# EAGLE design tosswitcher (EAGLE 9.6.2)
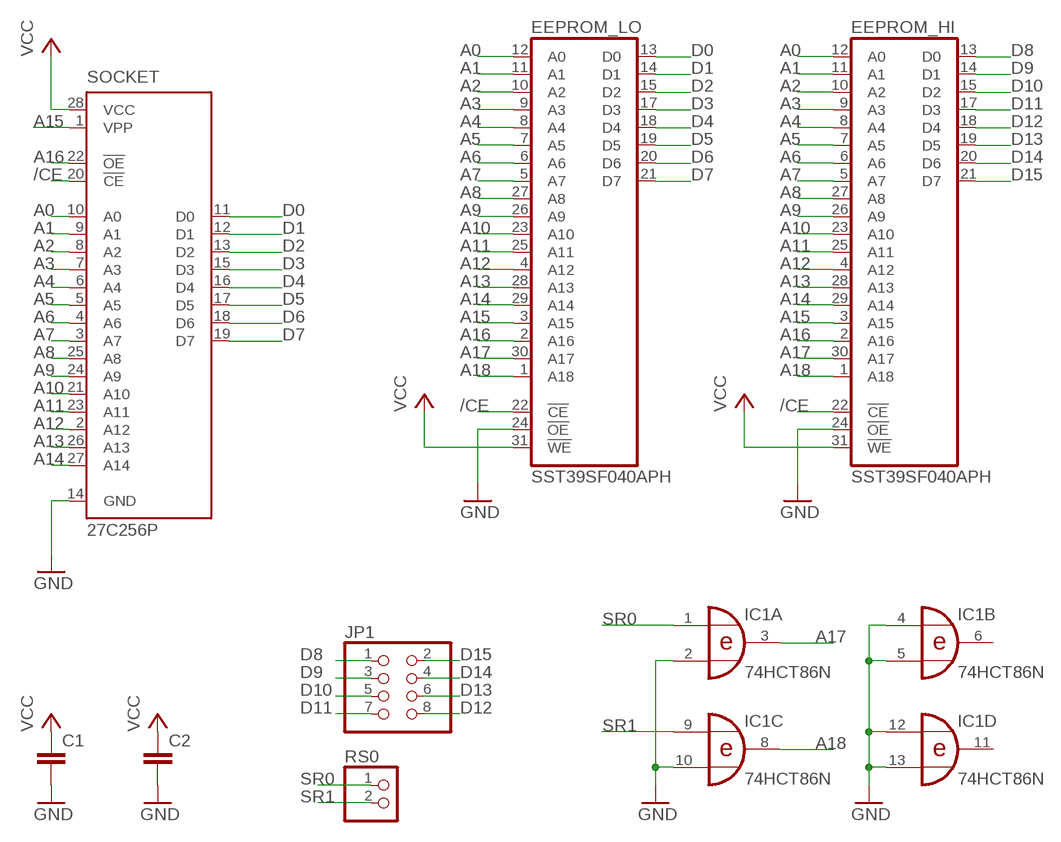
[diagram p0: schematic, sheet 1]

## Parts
C1  C2,5-3  [C2.5-3]
C2  C2,5-3  [C2.5-3]
EEPROM_HI  SST39SF040APH  [DIL32]
EEPROM_LO  SST39SF040APH  [DIL32]
IC1  74HCT86N  [DIL14]
JP1  PINHD-2X4/90  [2X04/90]
RS0  PINHD-1X2/90  [1X02/90]
SOCKET  27C256P  [DIL28-6]

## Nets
/CE: EEPROM_HI.22(!CE) EEPROM_LO.22(!CE) SOCKET.20(!CE)
A0: EEPROM_HI.12(A0) EEPROM_LO.12(A0) SOCKET.10(A0)
A1: EEPROM_HI.11(A1) EEPROM_LO.11(A1) SOCKET.9(A1)
A2: EEPROM_HI.10(A2) EEPROM_LO.10(A2) SOCKET.8(A2)
A3: EEPROM_HI.9(A3) EEPROM_LO.9(A3) SOCKET.7(A3)
A4: EEPROM_HI.8(A4) EEPROM_LO.8(A4) SOCKET.6(A4)
A5: EEPROM_HI.7(A5) EEPROM_LO.7(A5) SOCKET.5(A5)
A6: EEPROM_HI.6(A6) EEPROM_LO.6(A6) SOCKET.4(A6)
A7: EEPROM_HI.5(A7) EEPROM_LO.5(A7) SOCKET.3(A7)
A8: EEPROM_HI.27(A8) EEPROM_LO.27(A8) SOCKET.25(A8)
A9: EEPROM_HI.26(A9) EEPROM_LO.26(A9) SOCKET.24(A9)
A10: EEPROM_HI.23(A10) EEPROM_LO.23(A10) SOCKET.21(A10)
A11: EEPROM_HI.25(A11) EEPROM_LO.25(A11) SOCKET.23(A11)
A12: EEPROM_HI.4(A12) EEPROM_LO.4(A12) SOCKET.2(A12)
A13: EEPROM_HI.28(A13) EEPROM_LO.28(A13) SOCKET.26(A13)
A14: EEPROM_HI.29(A14) EEPROM_LO.29(A14) SOCKET.27(A14)
A15: EEPROM_HI.3(A15) EEPROM_LO.3(A15) SOCKET.1(VPP)
A16: EEPROM_HI.2(A16) EEPROM_LO.2(A16) SOCKET.22(!OE)
A17: EEPROM_HI.30(A17) EEPROM_LO.30(A17) IC1.3(A:O)
A18: EEPROM_HI.1(A18) EEPROM_LO.1(A18) IC1.8(C:O)
D0: EEPROM_LO.13(D0) SOCKET.11(D0)
D1: EEPROM_LO.14(D1) SOCKET.12(D1)
D2: EEPROM_LO.15(D2) SOCKET.13(D2)
D3: EEPROM_LO.17(D3) SOCKET.15(D3)
D4: EEPROM_LO.18(D4) SOCKET.16(D4)
D5: EEPROM_LO.19(D5) SOCKET.17(D5)
D6: EEPROM_LO.20(D6) SOCKET.18(D6)
D7: EEPROM_LO.21(D7) SOCKET.19(D7)
D8: EEPROM_HI.13(D0) JP1.1
D9: EEPROM_HI.14(D1) JP1.3
D10: EEPROM_HI.15(D2) JP1.5
D11: EEPROM_HI.17(D3) JP1.7
D12: EEPROM_HI.18(D4) JP1.8
D13: EEPROM_HI.19(D5) JP1.6
D14: EEPROM_HI.20(D6) JP1.4
D15: EEPROM_HI.21(D7) JP1.2
GND: C1.2 C2.2 EEPROM_HI.24(!OE) EEPROM_LO.24(!OE) IC1.2(A:I1) IC1.4(B:I0) IC1.5(B:I1) IC1.10(C:I1) IC1.12(D:I0) IC1.13(D:I1) SOCKET.14(GND)
SR0: IC1.1(A:I0) RS0.1
SR1: IC1.9(C:I0) RS0.2
VCC: C1.1 C2.1 EEPROM_HI.31(!WE) EEPROM_LO.31(!WE) SOCKET.28(VCC)
Unconnected: IC1.6(B:O) IC1.11(D:O)

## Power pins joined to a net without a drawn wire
GND: EEPROM_HI.16(GND) EEPROM_LO.16(GND) IC1.7(P:GND)
VCC: EEPROM_HI.32(VCC) EEPROM_LO.32(VCC) IC1.14(P:VCC)

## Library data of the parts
C1 C2 = capacitor-wima:C: CAPACITOR
EEPROM_HI EEPROM_LO = SST39SF040:SST39SF040A: 4 Mbit x8 Multi-Purpose Flash Source: http://www.sst.com/dotAsset/40782.pdf
IC1 = 74xx-eu:74*86: Quad 2-input EXCLUSIVE-OR (XOR) gate
JP1 = pinhead:PINHD-2X4: PIN HEADER
RS0 = pinhead:PINHD-1X2: PIN HEADER
SOCKET = socket:27*256: CMOS EPROM 256 K (32 K x 8), low voltage; MF: Arrow Electronics; MPN: M27C256B15F1; OC_FARNELL: 1125431; OC_NEWARK: 93K7335

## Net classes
0 default: clearance 0.205 mm

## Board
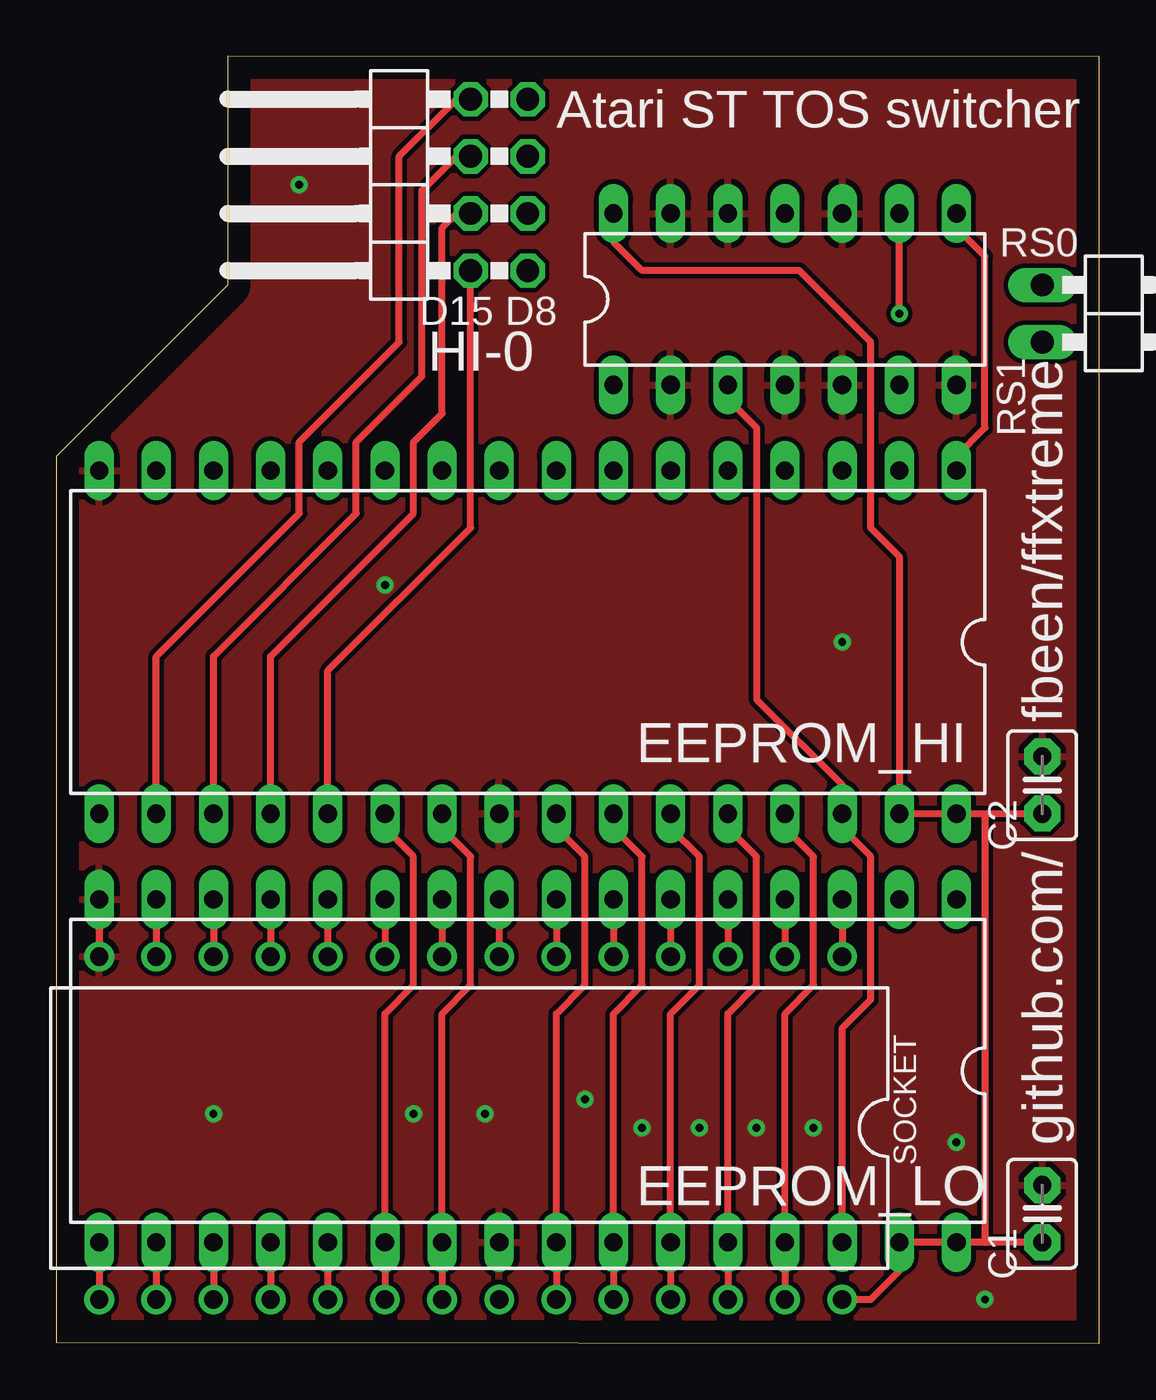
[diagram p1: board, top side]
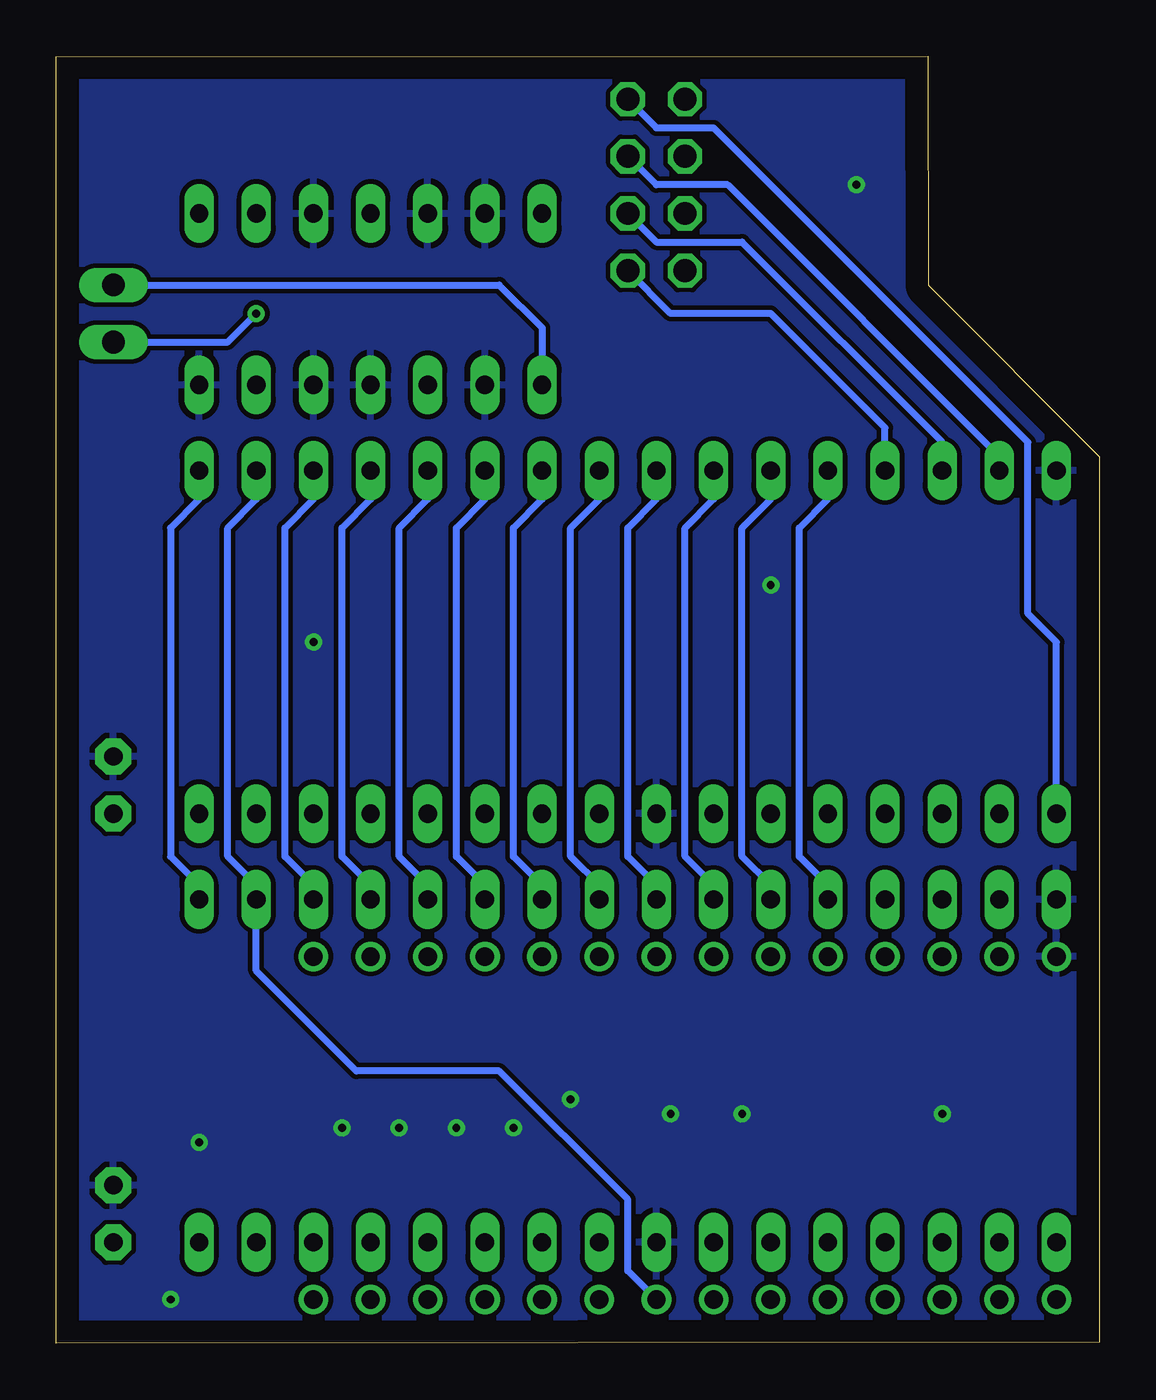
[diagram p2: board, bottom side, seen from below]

Size 46.35 x 57.19 mm. Coordinates in mm from the lower left corner, seen from the top.
Outline: 0,0.04 46.35,0 46.35,57.16 7.62,57.19 7.61,47.02 0,39.4 0,0.04
Copper layers (1*16): Top 0.035mm / dielectric 1.5mm / Bottom 0.035mm
Design rules "default": minimum track width 6mil, minimum drill 0.35mm, track to track 6mil, track to pad 6mil, pad to pad 6mil, via to via 6mil, smd to smd 6mil, copper to edge 40mil, drill to drill 6mil, minimum pad ring 10mil, minimum via ring 8mil, stop-mask expansion 4mil, vias tented up to drill 0mil, thermal gap 10mil

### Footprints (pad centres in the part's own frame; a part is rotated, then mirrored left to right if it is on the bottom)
C2.5-3 = drill 0.813 pad 1.6 octagon: 1 -1.27,0; 2 1.27,0
DIL32 = drill 0.813 long: 1 -19.05,-7.62; 2 -16.51,-7.62; 3 -13.97,-7.62; 4 -11.43,-7.62; 5 -8.89,-7.62; 6 -6.35,-7.62; 7 -3.81,-7.62; 8 -1.27,-7.62; 9 1.27,-7.62; 10 3.81,-7.62; 11 6.35,-7.62; 12 8.89,-7.62; 13 11.43,-7.62; 14 13.97,-7.62; 15 16.51,-7.62; 16 19.05,-7.62; 17 19.05,7.62; 18 16.51,7.62; 19 13.97,7.62; 20 11.43,7.62; 21 8.89,7.62; 22 6.35,7.62; 23 3.81,7.62; 24 1.27,7.62; 25 -1.27,7.62; 26 -3.81,7.62; 27 -6.35,7.62; 28 -8.89,7.62; 29 -11.43,7.62; 30 -13.97,7.62; 31 -16.51,7.62; 32 -19.05,7.62
DIL14 = drill 0.813 long: 1 -7.62,-3.81; 2 -5.08,-3.81; 3 -2.54,-3.81; 4 0,-3.81; 5 2.54,-3.81; 6 5.08,-3.81; 7 7.62,-3.81; 8 7.62,3.81; 9 5.08,3.81; 10 2.54,3.81; 11 0,3.81; 12 -2.54,3.81; 13 -5.08,3.81; 14 -7.62,3.81
2X04/90 = drill 1.016 octagon: 1 -3.81,-6.35; 2 -3.81,-3.81; 3 -1.27,-6.35; 4 -1.27,-3.81; 5 1.27,-6.35; 6 1.27,-3.81; 7 3.81,-6.35; 8 3.81,-3.81
1X02/90 = drill 1.016 long: 1 -1.27,-3.81; 2 1.27,-3.81
DIL28-6 = drill 0.813: 1 -16.51,-7.62; 2 -13.97,-7.62; 3 -11.43,-7.62; 4 -8.89,-7.62; 5 -6.35,-7.62; 6 -3.81,-7.62; 7 -1.27,-7.62; 8 1.27,-7.62; 9 3.81,-7.62; 10 6.35,-7.62; 11 8.89,-7.62; 12 11.43,-7.62; 13 13.97,-7.62; 14 16.51,-7.62; 15 16.51,7.62; 16 13.97,7.62; 17 11.43,7.62; 18 8.89,7.62; 19 6.35,7.62; 20 3.81,7.62; 21 1.27,7.62; 22 -1.27,7.62; 23 -3.81,7.62; 24 -6.35,7.62; 25 -8.89,7.62; 26 -11.43,7.62; 27 -13.97,7.62; 28 -16.51,7.62

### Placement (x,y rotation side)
C1  43.81,5.75 90 top
C2  43.81,24.8 90 top
EEPROM_HI  20.95,31.15 180 top
EEPROM_LO  20.95,12.1 180 top
IC1  32.38,46.39 0 top
JP1  14.61,51.47 90 top
RS0  47.62,45.76 270 top
SOCKET  18.41,9.56 180 top

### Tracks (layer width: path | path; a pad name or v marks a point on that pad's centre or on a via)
/CE
  Top 0.305: SOCKET.20 EEPROM_LO.22 14.61,14.64 15.88,15.91 15.88,21.63 14.61,22.9 EEPROM_HI.22
A0
  Top 0.305: EEPROM_LO.12 SOCKET.10
  Bottom 0.305: EEPROM_LO.12 12.06,20.36 13.34,21.63 13.34,36.23 12.06,37.5 EEPROM_HI.12
A1
  Top 0.305: EEPROM_LO.11 SOCKET.9
  Bottom 0.305: EEPROM_LO.11 14.61,20.36 15.88,21.63 15.88,36.23 14.61,37.5 EEPROM_HI.11
A2
  Top 0.305: EEPROM_LO.10 SOCKET.8
  Bottom 0.305: EEPROM_LO.10 17.14,20.36 18.41,21.63 18.41,36.23 17.14,37.5 EEPROM_HI.10
A3
  Top 0.305: EEPROM_LO.9 SOCKET.7
  Bottom 0.305: EEPROM_LO.9 19.68,20.36 20.95,21.63 20.95,36.23 19.68,37.5 EEPROM_HI.9
A4
  Top 0.305: EEPROM_LO.8 SOCKET.6
  Bottom 0.305: EEPROM_LO.8 22.23,20.36 23.5,21.63 23.5,36.23 22.23,37.5 EEPROM_HI.8
A5
  Top 0.305: EEPROM_LO.7 SOCKET.5
  Bottom 0.305: EEPROM_LO.7 24.77,20.36 26.04,21.63 26.04,36.23 24.77,37.5 EEPROM_HI.7
A6
  Top 0.305: EEPROM_LO.6 SOCKET.4
  Bottom 0.305: EEPROM_LO.6 27.3,20.36 28.57,21.63 28.57,36.23 27.3,37.5 EEPROM_HI.6
A7
  Top 0.305: EEPROM_LO.5 SOCKET.3
  Bottom 0.305: EEPROM_LO.5 29.84,20.36 31.11,21.63 31.11,36.23 29.84,37.5 EEPROM_HI.5
A8
  Top 0.305: SOCKET.25 EEPROM_LO.27 27.3,14.64 28.57,15.91 28.57,21.63 27.3,22.9 EEPROM_HI.27
A9
  Top 0.305: SOCKET.24 EEPROM_LO.26 24.77,14.64 26.04,15.91 26.04,21.63 24.77,22.9 EEPROM_HI.26
A10
  Top 0.305: SOCKET.21 EEPROM_LO.23 17.14,14.64 18.41,15.91 18.41,21.63 17.14,22.9 EEPROM_HI.23
A11
  Top 0.305: SOCKET.23 EEPROM_LO.25 22.23,14.64 23.5,15.91 23.5,21.63 22.23,22.9 EEPROM_HI.25
A12
  Top 0.305: EEPROM_LO.4 SOCKET.2
  Bottom 0.305: EEPROM_LO.4 32.38,20.36 33.66,21.63 33.66,36.23 32.38,37.5 EEPROM_HI.4
A13
  Top 0.305: SOCKET.26 EEPROM_LO.28 29.84,14.64 31.11,15.91 31.11,21.63 29.84,22.9 EEPROM_HI.28
A14
  Top 0.305: SOCKET.27 EEPROM_LO.29 32.38,14.64 33.66,15.91 33.66,21.63 32.38,22.9 EEPROM_HI.29
A15
  Top 0.305: EEPROM_LO.3 SOCKET.1
  Bottom 0.305: EEPROM_LO.3 34.92,20.36 36.2,21.63 36.2,36.23 34.92,37.5 EEPROM_HI.3
A16
  Bottom 0.305: SOCKET.22 20.95,3.21 20.95,6.39 26.67,12.1 33.02,12.1 37.47,16.55 EEPROM_LO.2 37.47,20.36 38.73,21.63 38.73,36.23 37.47,37.5 EEPROM_HI.2
A17
  Top 0.305: EEPROM_LO.30 34.92,14.01 36.2,15.28 36.2,21.63 34.92,22.9 EEPROM_HI.30 34.92,24.8 31.11,28.61 31.11,40.68 29.84,41.95 IC1.3
A18
  Top 0.305: EEPROM_HI.1 40.01,39.41 41.27,40.68 41.27,48.3 40.01,49.57 IC1.8
  Bottom 0.305: EEPROM_HI.1 40.01,37.5 41.27,36.23 41.27,21.63 40.01,20.36 EEPROM_LO.1
D0
  Top 0.305: EEPROM_LO.13 SOCKET.11
D1
  Top 0.305: EEPROM_LO.14 SOCKET.12
D2
  Top 0.305: EEPROM_LO.15 SOCKET.13
D3
  Top 0.305: EEPROM_LO.17 SOCKET.15
D4
  Top 0.305: EEPROM_LO.18 SOCKET.16
D5
  Top 0.305: EEPROM_LO.19 SOCKET.17
D6
  Top 0.305: EEPROM_LO.20 SOCKET.18
D7
  Top 0.305: EEPROM_LO.21 SOCKET.19
D8
  Bottom 0.305: EEPROM_HI.13 9.53,40.68 14.61,45.76 19.05,45.76 JP1.1
D9
  Bottom 0.305: EEPROM_HI.14 6.99,40.04 15.88,48.93 19.68,48.93 JP1.3
D10
  Bottom 0.305: EEPROM_HI.15 4.45,39.41 16.51,51.47 19.68,51.47 JP1.5
D11
  Bottom 0.305: EEPROM_HI.17 1.91,31.15 3.17,32.42 3.17,40.04 17.14,54.01 19.68,54.01 JP1.7
D12
  Top 0.305: EEPROM_HI.18 4.45,30.52 10.79,36.87 10.79,40.04 15.24,44.49 15.24,52.74 17.78,55.28 JP1.8
D13
  Top 0.305: EEPROM_HI.19 6.99,30.52 13.34,36.87 13.34,40.04 16.26,42.96 16.26,51.22 17.78,52.74 JP1.6
D14
  Top 0.305: EEPROM_HI.20 9.53,30.52 15.88,36.87 15.88,40.04 17.14,41.31 17.14,49.57 17.78,50.2 JP1.4
D15
  Top 0.305: EEPROM_HI.21 12.06,29.88 18.41,36.23 JP1.2
GND  (via drill 0.35)
  Top 0.305: EEPROM_LO.16 SOCKET.14
  other vias: 40.01,8.93 41.27,1.94 6.99,10.2 19.05,10.2 15.88,10.2 23.5,10.83 26.04,9.56 28.57,9.56 31.11,9.56 33.66,9.56 14.61,33.69 34.92,31.15 10.79,51.47
  pour Top: 7.62,57.19 46.35,57.19 46.35,0.04 0,0.04 0,39.41 7.62,47.03
  pour Bottom: 7.62,57.19 46.35,57.19 46.35,0.04 0,0.04 0,39.41 7.62,47.03
SR0
  Bottom 0.305: RS0.1 26.67,47.03 24.77,45.12 IC1.1
SR1  (via drill 0.35)
  Top 0.305: v37.47,45.76 IC1.9
  Bottom 0.305: RS0.2 38.73,44.49 v37.47,45.76
VCC
  Top 0.305: SOCKET.28 36.2,1.94 37.47,3.21 EEPROM_LO.31 EEPROM_LO.32 41.27,4.48 | 41.27,23.53 EEPROM_HI.32 EEPROM_HI.31 37.47,34.96 36.2,36.23 36.2,44.49 33.02,47.66 26.04,47.66 24.77,48.93 IC1.14 | 41.27,23.53 C2.1 | C1.1 41.27,4.48 | 41.27,23.53 41.27,4.48

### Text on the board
tNames: Atari ST TOS switcher | D15 | D8 | HI-0 | RS1 | fbeen/ffxtreme | github.com/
